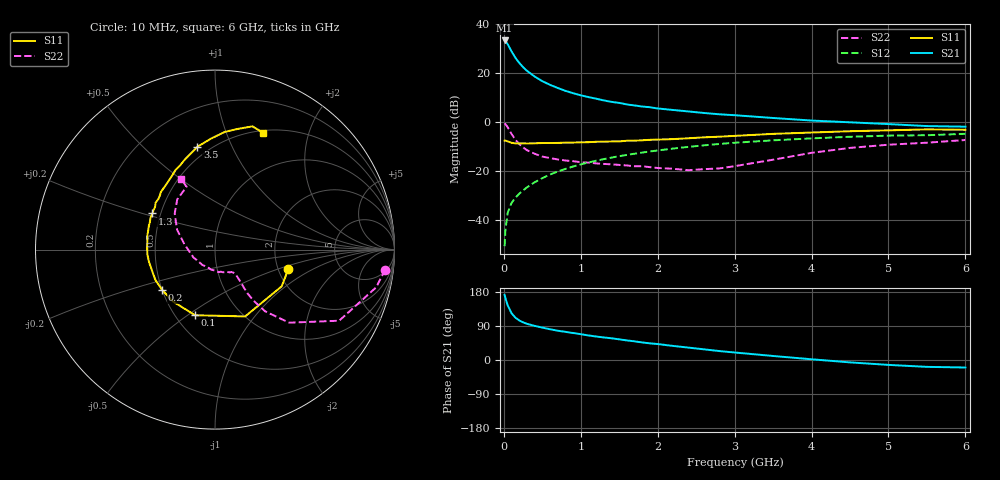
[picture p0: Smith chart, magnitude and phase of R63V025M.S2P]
! SIEMENS Small Signal Semiconductors
! BFR193
! Si NPN RF Bipolar Junction Transistor in SOT23
! VCE = 3 V  IC = 25 mA
! Common Emitter S-Parameters:  May  1996
# GHz  S  MA  R  50
!  f  S11  S21  S12  S22
! GHz  MAG  ANG  MAG  ANG  MAG  ANG  MAG  ANG
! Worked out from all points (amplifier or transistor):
!   36 points, 10 MHz to 6 GHz, reference 50 ohm
!   highest |S21| = 33.3 dB at 10 MHz (marker M1)
!   |S21| within 3 dB of that: start of sweep to 75.43 MHz
!   unconditionally stable (mu >= 1): 496.2 MHz to 1.854 GHz; 1.984 GHz to 2.019 GHz
!   at 250 MHz: K = 0.88, MSG = 25.1 dB, |S12| = -27.7 dB
!   at 1.4 GHz: K = 1.03, MAG = 10.4 dB, |S12| = -14.4 dB
!   at 6 GHz: K = 0.95, MSG = 1.5 dB, |S12| = -4.7 dB
!   S11 on the Smith chart (normalised r, x): 10 MHz: 2.27, -0.60; 100 MHz: 0.62, -0.54; 200 MHz: 0.50, -0.26; 1.3 GHz: 0.45, +0.22; 3.5 GHz: 0.43, +0.75; 6 GHz: 0.53, +1.36
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0.01  0.4229 -15.0  46.46 171.8  0.003 84.6  0.9551 -6.7
0.02  0.4241 -28.9  45.28 163.8  0.0063 79.1  0.922 -13.2
0.05  0.4085 -65.7  38.99 144.2  0.0143 70.6  0.7972 -29.8
0.1  0.3821 -106.8  27.91 123.5  0.0228 64.9  0.5799 -44.6
0.15  0.3722 -128.9  20.67 111.7  0.029 63.9  0.4434 -50.9
0.2  0.3705 -142.9  16.27 104.5  0.0351 65.9  0.3611 -52.8
0.25  0.3727 -152.7  13.27 99.4  0.0411 66.8  0.3079 -53.4
0.3  0.37 -159.1  11.19 95.6  0.0472 68.6  0.2708 -52.9
0.4  0.3739 -169.2  8.565 90.1  0.06 69.7  0.2294 -51.6
0.5  0.3781 -176.1  6.889 85.5  0.0728 70.5  0.2003 -50.8
0.6  0.3785 177.2  5.803 81.2  0.0863 70.6  0.1868 -50.4
0.7  0.3802 172.9  5.002 77.3  0.0993 70.2  0.1751 -50.6
0.8  0.3849 168.7  4.373 74.3  0.1123 69.1  0.1668 -51.0
1.1  0.3935 157.4  3.261 64.8  0.1521 66.9  0.1511 -57.1
1.3  0.4028 150.0  2.791 59.5  0.1784 64.5  0.142 -61.6
1.8  0.4302 135.5  2.094 46.3  0.2421 57.8  0.1277 -79.2
2.2  0.4552 126.1  1.783 37.1  0.2919 52.3  0.1131 -101.2
2.8  0.5094 112.2  1.457 23.6  0.362 43.3  0.1149 -147.5
3.5  0.5813 99.7  1.224 10.6  0.4294 32.3  0.1731 170.0
4.5  0.6583 85.2  1 -6.3  0.5073 18.1  0.3011 138.2
5.5  0.7177 73.1  0.838 -18.1  0.5461 3.9  0.3843 114.3
6  0.7038 67.6  0.815 -19.8  0.5823 -0.3  0.4361 115.7
